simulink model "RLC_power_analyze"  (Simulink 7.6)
settings: Solver=ode23tb  StartTime=0.0  StopTime=0.6  RelTol=1e-3
InitFcn:
  | % valeurs de R, L et C
  | R=3.3;
  | L=100e-3;
  | C=1e-3;
libraries: powerlib x8

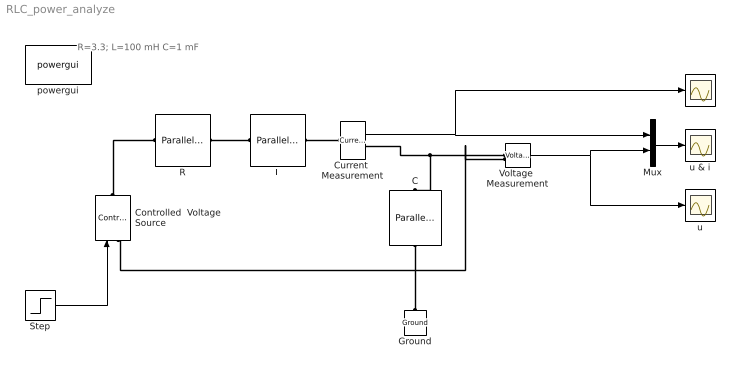
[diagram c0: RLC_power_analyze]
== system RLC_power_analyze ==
  note: R=3.3; L=100 mH C=1 mF
  C : powerlib/Elements/Parallel RLC Branch  DialogController=POWERSYS.PowerSysDialog  PhysicalDomain=powersysdomain  SubClassName=unknown  LeftPortType=p1  RightPortType=p1  LConnTagsString=a  RConnTagsString=__new0  BranchType=C  Resistance=1e-3  Inductance=1e-3  SetiL0=off  InitialCurrent=0  Capacitance=C  Setx0=off  InitialVoltage=0  Measurements=None
  Controlled  Voltage Source : powerlib/Electrical Sources/Controlled Voltage Source  DialogController=POWERSYS.PowerSysDialog  SystemSampleTime=-1  Initialize=on  Source_Type=AC  Amplitude=0  Phase=0  Frequency=0  Measurements=None
  Current  Measurement : powerlib/Measurements/Current Measurement  DialogController=POWERSYS.PowerSysDialog  SystemSampleTime=-1  PhasorSimulation=off  OutputType=Complex  PSBequivalent=0
  Ground : powerlib/Elements/Ground  DialogController=POWERSYS.PowerSysDialog  PhysicalDomain=powersysdomain  SubClassName=unknown  LeftPortType=p1  RightPortType=p1  LConnTagsString=a
  L : powerlib/Elements/Parallel RLC Branch  DialogController=POWERSYS.PowerSysDialog  PhysicalDomain=powersysdomain  SubClassName=unknown  LeftPortType=p1  RightPortType=p1  LConnTagsString=a  RConnTagsString=__new0  BranchType=L  Resistance=1e-3  Inductance=L  SetiL0=on  InitialCurrent=10e-3  Capacitance=1e-6  Setx0=off  InitialVoltage=0  Measurements=None
  Mux : Mux  Inputs=2
  R : powerlib/Elements/Parallel RLC Branch  DialogController=POWERSYS.PowerSysDialog  PhysicalDomain=powersysdomain  SubClassName=unknown  LeftPortType=p1  RightPortType=p1  LConnTagsString=a  RConnTagsString=__new0  BranchType=R  Resistance=R  Inductance=1e-3  SetiL0=off  InitialCurrent=0  Capacitance=1e-6  Setx0=off  InitialVoltage=0  Measurements=None
  Step : Step  Time=0.1  SampleTime=0
  Voltage  Measurement : powerlib/Measurements/Voltage Measurement  DialogController=POWERSYS.PowerSysDialog  SystemSampleTime=-1  PhasorSimulation=off  OutputType=Complex  PSBequivalent=0
  i : Scope
  powergui : powerlib/powergui  Priority=1  SystemSampleTime=-1  SimulationMode=Continuous  SampleTime=50e-6  frequency=60  SPID=off  DisableSnubberDevices=off  DisableRonSwitches=off  DisableVfSwitches=off  SwTol=0  Interpol=off  frequencyindice=0  echomessages=off  HookPort=off  DisplayEquations=off  FunctionMessages=off  EnableUseOfTLC=off  x0status=blocks  RestoreLinks=warning  ResistiveCurrentMeasurement=off  Ylog=off  Xlog=on  ShowGrid=off  save=off  variable=ZData  ZoomFFT=off  StartTime=0.0  cycles=1  DisplayStyle=1  FreqAxis=off  MaxFrequency=1000  frequencyindicesteady=1  display=off  methode=off
  u : Scope
  u & i : Scope
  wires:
  Step/1 -> Controlled  Voltage Source/1
  Voltage  Measurement/1 -> Mux/2, u/1
  Current  Measurement/1 -> Mux/1, i/1
  Mux/1 -> u & i/1
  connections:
  R/RConn1 -- L/LConn1
  Voltage  Measurement/LConn1 -- C/LConn1 -- Current  Measurement/RConn1
  C/RConn1 -- Ground/LConn1 -- Controlled  Voltage Source/LConn1 -- Voltage  Measurement/LConn2
  Controlled  Voltage Source/RConn1 -- R/LConn1
  L/RConn1 -- Current  Measurement/LConn1
